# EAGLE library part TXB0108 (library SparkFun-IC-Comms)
8-Bit Bi-Directional Level Shifter 1.2V-3.6V (VCCA) to 1.65V-5.5V (VCCB) bi-directional level shifter with auto direction sensing. Max data rate - VCCA 1.2V: 20Mbps (50ns), VCCA 3.3V: 100Mbps (10ns) Digikey: 296-27217-1-ND (20-UFDFN) SparkFun Products SparkFun GPS Logger Shield (GPS-13750) SparkFun Block for Intel® Edison - microSD (DEV-13041) SparkFun Block for Intel® Edison - Dual H-Bridge (DEV-13043) SparkFun Block for Intel® Edison - GPIO (DEV-13038) SparkFun Block for Intel® Edison - Raspberry Pi B (DEV-13044)
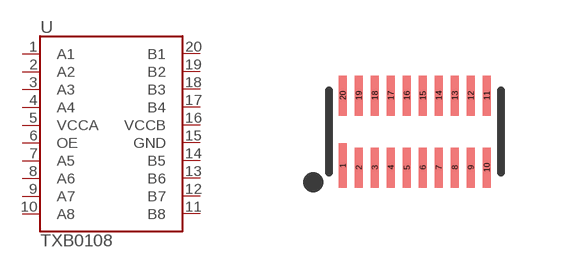
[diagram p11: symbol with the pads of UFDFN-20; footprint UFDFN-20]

Designator prefix U

## TXB0108 (PROD_ID: IC-12292; VALUE: TXB0108DQSR)  [UFDFN-20]
1  A1
2  A2
3  A3
4  A4
5  VCCA
6  OE
7  A5
8  A6
9  A7
10  A8
11  B8
12  B7
13  B6
14  B5
15  GND
16  VCCB
17  B4
18  B3
19  B2
20  B1

## Footprint UFDFN-20 (pad centres in mm)
UFDFN-20 Specifications: Pin count: 20 Example device(s): TXB0108
smd 0.2 x 1.1: 1 -1.8,-0.85
smd 0.2 x 1: 2 -1.4,-0.9; 3 -1,-0.9; 4 -0.6,-0.9; 5 -0.2,-0.9; 6 0.2,-0.9; 7 0.6,-0.9; 8 1,-0.9; 9 1.4,-0.9; 10 1.8,-0.9; 11 1.8,0.9; 12 1.4,0.9; 13 1,0.9; 14 0.6,0.9; 15 0.2,0.9; 16 -0.2,0.9; 17 -0.6,0.9; 18 -1,0.9; 19 -1.4,0.9; 20 -1.8,0.9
